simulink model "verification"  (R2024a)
settings: Solver=ode4  StartTime=0.0  StopTime=20  FixedStep=0.2  RelTol=1e-3

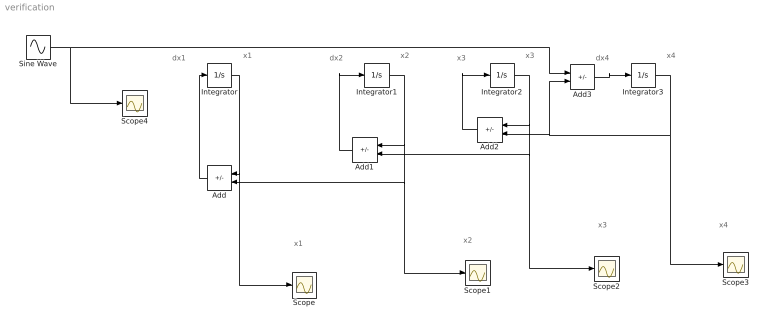
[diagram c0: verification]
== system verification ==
  note: x3
  note: x2
  note: x1
  note: x1
  note: dx1
  note: x2
  note: dx2
  note: x3
  note: x3
  note: x4
  note: dx4
  note: x4
  Add : Sum  Inputs=-+
  Add1 : Sum  Inputs=-+
  Add2 : Sum  Inputs=-+
  Add3 : Sum  Inputs=+-
  Integrator{,1..3} (4 alike) : Integrator
  Scope{,1..4} (5 alike) : Scope
  Sine Wave : Sin  Frequency=2*pi  SampleTime=0
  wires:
  Integrator1/1 -> Scope1/1, Add/2, Add1/1
  Integrator2/1 -> Add2/1, Scope2/1, Add1/2
  Integrator3/1 -> Scope3/1, Add3/2, Add2/2
  Integrator/1 -> Scope/1, Add/1
  Add/1 -> Integrator/1
  Add1/1 -> Integrator1/1
  Add2/1 -> Integrator2/1
  Add3/1 -> Integrator3/1
  Sine Wave/1 -> Scope4/1, Add3/1
